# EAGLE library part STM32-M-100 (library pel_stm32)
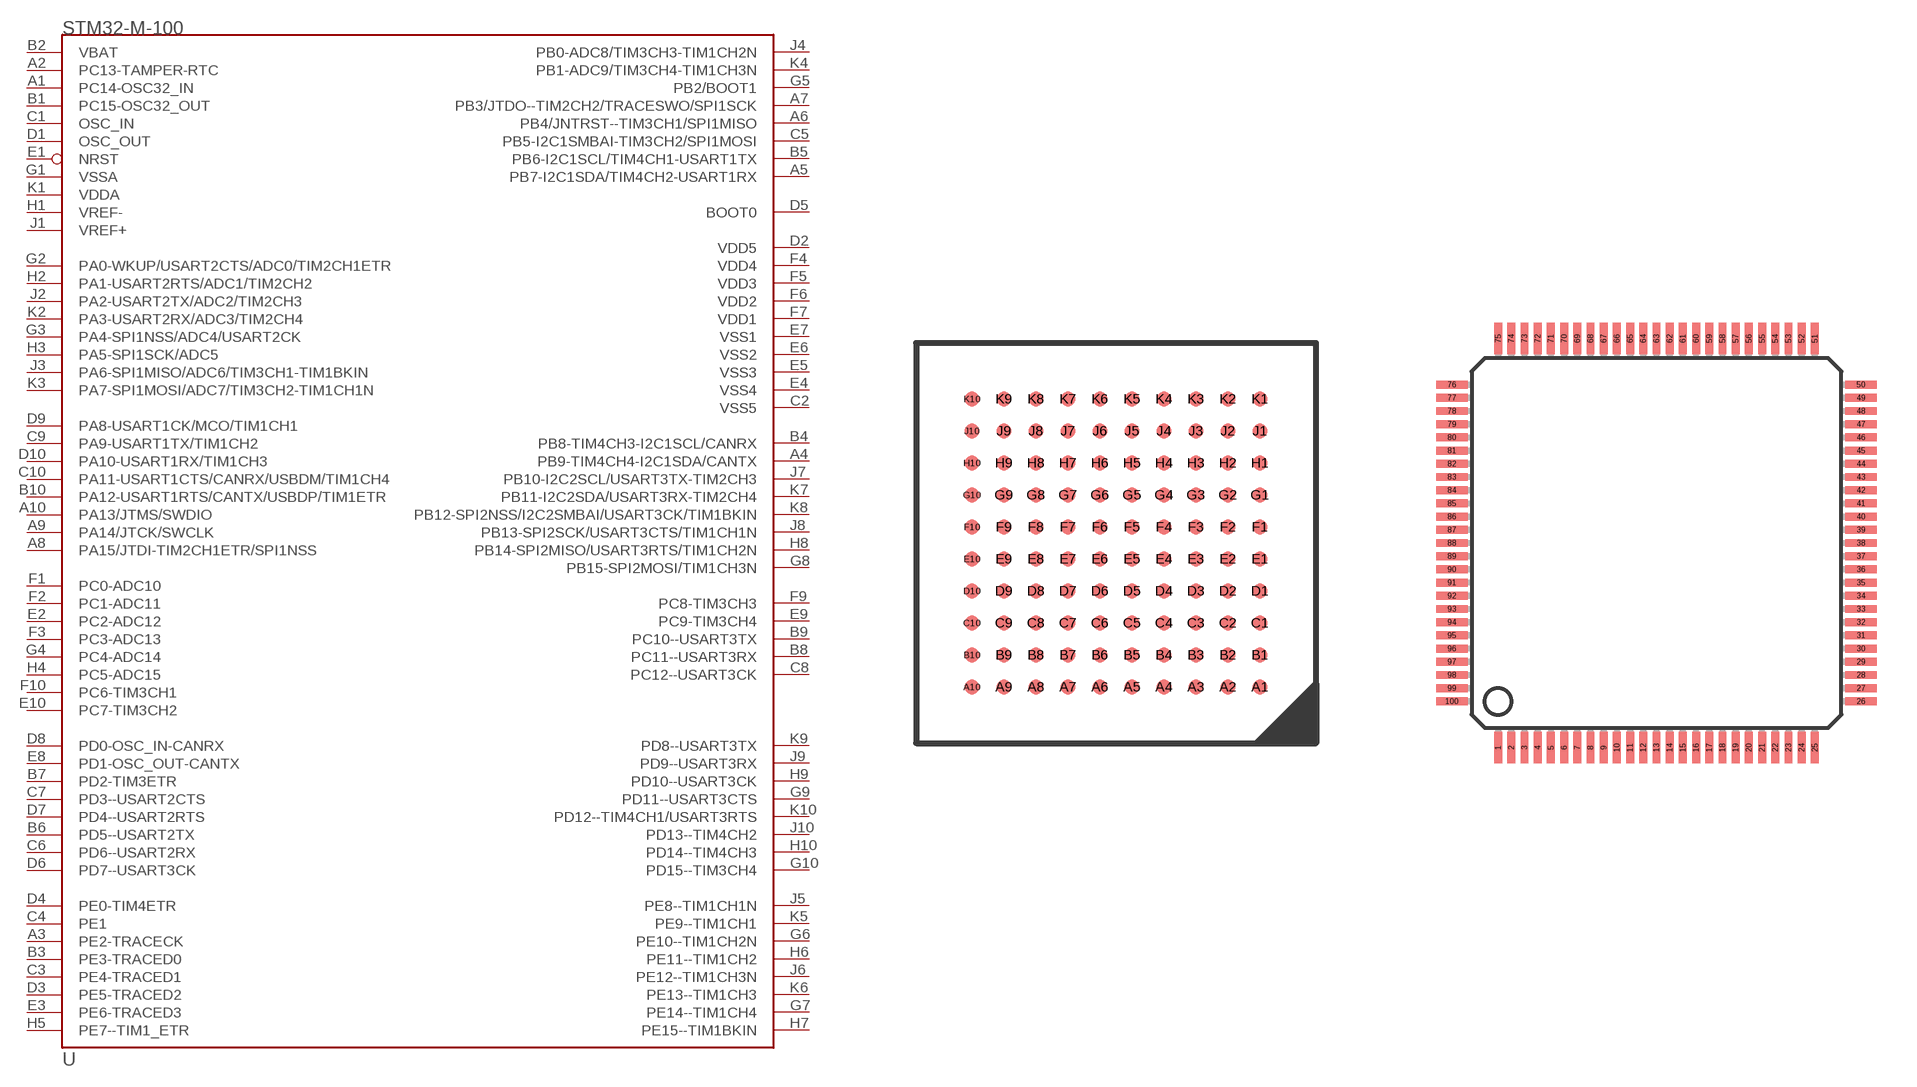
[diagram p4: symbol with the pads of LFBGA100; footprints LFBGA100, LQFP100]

Designator prefix U

## STM32-M-100-LFBGA  [LFBGA100]
A1  PC14-OSC32_IN
A2  PC13-TAMPER-RTC
A3  PE2-TRACECK
A4  PB9-TIM4CH4-I2C1SDA/CANTX
A5  PB7-I2C1SDA/TIM4CH2-USART1RX
A6  PB4/JNTRST--TIM3CH1/SPI1MISO
A7  PB3/JTDO--TIM2CH2/TRACESWO/SPI1SCK
A8  PA15/JTDI-TIM2CH1ETR/SPI1NSS
A9  PA14/JTCK/SWCLK
A10  PA13/JTMS/SWDIO
B1  PC15-OSC32_OUT
B2  VBAT  sup
B3  PE3-TRACED0
B4  PB8-TIM4CH3-I2C1SCL/CANRX
B5  PB6-I2C1SCL/TIM4CH1-USART1TX
B6  PD5--USART2TX
B7  PD2-TIM3ETR
B8  PC11--USART3RX
B9  PC10--USART3TX
B10  PA12-USART1RTS/CANTX/USBDP/TIM1ETR
C1  OSC_IN  in
C2  VSS5
C3  PE4-TRACED1
C4  PE1
C5  PB5-I2C1SMBAI-TIM3CH2/SPI1MOSI
C6  PD6--USART2RX
C7  PD3--USART2CTS
C8  PC12--USART3CK
C9  PA9-USART1TX/TIM1CH2
C10  PA11-USART1CTS/CANRX/USBDM/TIM1CH4
D1  OSC_OUT  out
D2  VDD5
D3  PE5-TRACED2
D4  PE0-TIM4ETR
D5  BOOT0  in
D6  PD7--USART3CK
D7  PD4--USART2RTS
D8  PD0-OSC_IN-CANRX
D9  PA8-USART1CK/MCO/TIM1CH1
D10  PA10-USART1RX/TIM1CH3
E1  NRST
E2  PC2-ADC12
E3  PE6-TRACED3
E4  VSS4
E5  VSS3  sup
E6  VSS2  sup
E7  VSS1  sup
E8  PD1-OSC_OUT-CANTX
E9  PC9-TIM3CH4
E10  PC7-TIM3CH2
F1  PC0-ADC10
F2  PC1-ADC11
F3  PC3-ADC13
F4  VDD4
F5  VDD3  sup
F6  VDD2  sup
F7  VDD1  sup
F9  PC8-TIM3CH3
F10  PC6-TIM3CH1
G1  VSSA  sup
G2  PA0-WKUP/USART2CTS/ADC0/TIM2CH1ETR
G3  PA4-SPI1NSS/ADC4/USART2CK
G4  PC4-ADC14
G5  PB2/BOOT1
G6  PE10--TIM1CH2N
G7  PE14--TIM1CH4
G8  PB15-SPI2MOSI/TIM1CH3N
G9  PD11--USART3CTS
G10  PD15--TIM3CH4
H1  VREF-
H2  PA1-USART2RTS/ADC1/TIM2CH2
H3  PA5-SPI1SCK/ADC5
H4  PC5-ADC15
H5  PE7--TIM1_ETR
H6  PE11--TIM1CH2
H7  PE15--TIM1BKIN
H8  PB14-SPI2MISO/USART3RTS/TIM1CH2N
H9  PD10--USART3CK
H10  PD14--TIM4CH3
J1  VREF+
J2  PA2-USART2TX/ADC2/TIM2CH3
J3  PA6-SPI1MISO/ADC6/TIM3CH1-TIM1BKIN
J4  PB0-ADC8/TIM3CH3-TIM1CH2N
J5  PE8--TIM1CH1N
J6  PE12--TIM1CH3N
J7  PB10-I2C2SCL/USART3TX-TIM2CH3
J8  PB13-SPI2SCK/USART3CTS/TIM1CH1N
J9  PD9--USART3RX
J10  PD13--TIM4CH2
K1  VDDA  sup
K2  PA3-USART2RX/ADC3/TIM2CH4
K3  PA7-SPI1MOSI/ADC7/TIM3CH2-TIM1CH1N
K4  PB1-ADC9/TIM3CH4-TIM1CH3N
K5  PE9--TIM1CH1
K6  PE13--TIM1CH3
K7  PB11-I2C2SDA/USART3RX-TIM2CH4
K8  PB12-SPI2NSS/I2C2SMBAI/USART3CK/TIM1BKIN
K9  PD8--USART3TX
K10  PD12--TIM4CH1/USART3RTS

## STM32-M-100-LQFP  [LQFP100]
1  PE2-TRACECK
2  PE3-TRACED0
3  PE4-TRACED1
4  PE5-TRACED2
5  PE6-TRACED3
6  VBAT  sup
7  PC13-TAMPER-RTC
8  PC14-OSC32_IN
9  PC15-OSC32_OUT
10  VSS5
11  VDD5
12  OSC_IN  in
13  OSC_OUT  out
14  NRST
15  PC0-ADC10
16  PC1-ADC11
17  PC2-ADC12
18  PC3-ADC13
19  VSSA  sup
20  VREF-
21  VREF+
22  VDDA  sup
23  PA0-WKUP/USART2CTS/ADC0/TIM2CH1ETR
24  PA1-USART2RTS/ADC1/TIM2CH2
25  PA2-USART2TX/ADC2/TIM2CH3
26  PA3-USART2RX/ADC3/TIM2CH4
27  VSS4
28  VDD4
29  PA4-SPI1NSS/ADC4/USART2CK
30  PA5-SPI1SCK/ADC5
31  PA6-SPI1MISO/ADC6/TIM3CH1-TIM1BKIN
32  PA7-SPI1MOSI/ADC7/TIM3CH2-TIM1CH1N
33  PC4-ADC14
34  PC5-ADC15
35  PB0-ADC8/TIM3CH3-TIM1CH2N
36  PB1-ADC9/TIM3CH4-TIM1CH3N
37  PB2/BOOT1
38  PE7--TIM1_ETR
39  PE8--TIM1CH1N
40  PE9--TIM1CH1
41  PE10--TIM1CH2N
42  PE11--TIM1CH2
43  PE12--TIM1CH3N
44  PE13--TIM1CH3
45  PE14--TIM1CH4
46  PE15--TIM1BKIN
47  PB10-I2C2SCL/USART3TX-TIM2CH3
48  PB11-I2C2SDA/USART3RX-TIM2CH4
49  VSS1  sup
50  VDD1  sup
51  PB12-SPI2NSS/I2C2SMBAI/USART3CK/TIM1BKIN
52  PB13-SPI2SCK/USART3CTS/TIM1CH1N
53  PB14-SPI2MISO/USART3RTS/TIM1CH2N
54  PB15-SPI2MOSI/TIM1CH3N
55  PD8--USART3TX
56  PD9--USART3RX
57  PD10--USART3CK
58  PD11--USART3CTS
59  PD12--TIM4CH1/USART3RTS
60  PD13--TIM4CH2
61  PD14--TIM4CH3
62  PD15--TIM3CH4
63  PC6-TIM3CH1
64  PC7-TIM3CH2
65  PC8-TIM3CH3
66  PC9-TIM3CH4
67  PA8-USART1CK/MCO/TIM1CH1
68  PA9-USART1TX/TIM1CH2
69  PA10-USART1RX/TIM1CH3
70  PA11-USART1CTS/CANRX/USBDM/TIM1CH4
71  PA12-USART1RTS/CANTX/USBDP/TIM1ETR
72  PA13/JTMS/SWDIO
74  VSS2  sup
75  VDD2  sup
76  PA14/JTCK/SWCLK
77  PA15/JTDI-TIM2CH1ETR/SPI1NSS
78  PC10--USART3TX
79  PC11--USART3RX
80  PC12--USART3CK
81  PD0-OSC_IN-CANRX
82  PD1-OSC_OUT-CANTX
83  PD2-TIM3ETR
84  PD3--USART2CTS
85  PD4--USART2RTS
86  PD5--USART2TX
87  PD6--USART2RX
88  PD7--USART3CK
89  PB3/JTDO--TIM2CH2/TRACESWO/SPI1SCK
90  PB4/JNTRST--TIM3CH1/SPI1MISO
91  PB5-I2C1SMBAI-TIM3CH2/SPI1MOSI
92  PB6-I2C1SCL/TIM4CH1-USART1TX
93  PB7-I2C1SDA/TIM4CH2-USART1RX
94  BOOT0  in
95  PB8-TIM4CH3-I2C1SCL/CANRX
96  PB9-TIM4CH4-I2C1SDA/CANTX
97  PE0-TIM4ETR
98  PE1
99  VSS3  sup
100  VDD3  sup

## Footprint LFBGA100 (pad centres in mm)
smd 0.37 x 0.37: A1 3.6,-3.6; A2 2.8,-3.6; A3 2,-3.6; A4 1.2,-3.6; A5 0.4,-3.6; A6 -0.4,-3.6; A7 -1.2,-3.6; A8 -2,-3.6; A9 -2.8,-3.6; A10 -3.6,-3.6; B1 3.6,-2.8; B2 2.8,-2.8; B3 2,-2.8; B4 1.2,-2.8; B5 0.4,-2.8; B6 -0.4,-2.8; B7 -1.2,-2.8; B8 -2,-2.8; B9 -2.8,-2.8; B10 -3.6,-2.8; C1 3.6,-2; C2 2.8,-2; C3 2,-2; C4 1.2,-2; C5 0.4,-2; C6 -0.4,-2; C7 -1.2,-2; C8 -2,-2; C9 -2.8,-2; C10 -3.6,-2; D1 3.6,-1.2; D2 2.8,-1.2; D3 2,-1.2; D4 1.2,-1.2; D5 0.4,-1.2; D6 -0.4,-1.2; D7 -1.2,-1.2; D8 -2,-1.2; D9 -2.8,-1.2; D10 -3.6,-1.2; E1 3.6,-0.4; E2 2.8,-0.4; E3 2,-0.4; E4 1.2,-0.4; E5 0.4,-0.4; E6 -0.4,-0.4; E7 -1.2,-0.4; E8 -2,-0.4; E9 -2.8,-0.4; E10 -3.6,-0.4; F1 3.6,0.4; F2 2.8,0.4; F3 2,0.4; F4 1.2,0.4; F5 0.4,0.4; F6 -0.4,0.4; F7 -1.2,0.4; F8 -2,0.4; F9 -2.8,0.4; F10 -3.6,0.4; G1 3.6,1.2; G2 2.8,1.2; G3 2,1.2; G4 1.2,1.2; G5 0.4,1.2; G6 -0.4,1.2; G7 -1.2,1.2; G8 -2,1.2; G9 -2.8,1.2; G10 -3.6,1.2; H1 3.6,2; H2 2.8,2; H3 2,2; H4 1.2,2; H5 0.4,2; H6 -0.4,2; H7 -1.2,2; H8 -2,2; H9 -2.8,2; H10 -3.6,2; J1 3.6,2.8; J2 2.8,2.8; J3 2,2.8; J4 1.2,2.8; J5 0.4,2.8; J6 -0.4,2.8; J7 -1.2,2.8; J8 -2,2.8; J9 -2.8,2.8; J10 -3.6,2.8; K1 3.6,3.6; K2 2.8,3.6; K3 2,3.6; K4 1.2,3.6; K5 0.4,3.6; K6 -0.4,3.6; K7 -1.2,3.6; K8 -2,3.6; K9 -2.8,3.6; K10 -3.6,3.6

## Footprint LQFP100 (pad centres in mm)
smd 0.3 x 1.2: 1 -6,-7.75; 2 -5.5,-7.75; 3 -5,-7.75; 4 -4.5,-7.75; 5 -4,-7.75; 6 -3.5,-7.75; 7 -3,-7.75; 8 -2.5,-7.75; 9 -2,-7.75; 10 -1.5,-7.75; 11 -1,-7.75; 12 -0.5,-7.75; 13 0,-7.75; 14 0.5,-7.75; 15 1,-7.75; 16 1.5,-7.75; 17 2,-7.75; 18 2.5,-7.75; 19 3,-7.75; 20 3.5,-7.75; 21 4,-7.75; 22 4.5,-7.75; 23 5,-7.75; 24 5.5,-7.75; 25 6,-7.75; 51 6,7.75; 52 5.5,7.75; 53 5,7.75; 54 4.5,7.75; 55 4,7.75; 56 3.5,7.75; 57 3,7.75; 58 2.5,7.75; 59 2,7.75; 60 1.5,7.75; 61 1,7.75; 62 0.5,7.75; 63 0,7.75; 64 -0.5,7.75; 65 -1,7.75; 66 -1.5,7.75; 67 -2,7.75; 68 -2.5,7.75; 69 -3,7.75; 70 -3.5,7.75; 71 -4,7.75; 72 -4.5,7.75; 73 -5,7.75; 74 -5.5,7.75; 75 -6,7.75
smd 1.2 x 0.3: 26 7.75,-6; 27 7.75,-5.5; 28 7.75,-5; 29 7.75,-4.5; 30 7.75,-4; 31 7.75,-3.5; 32 7.75,-3; 33 7.75,-2.5; 34 7.75,-2; 35 7.75,-1.5; 36 7.75,-1; 37 7.75,-0.5; 38 7.75,0; 39 7.75,0.5; 40 7.75,1; 41 7.75,1.5; 42 7.75,2; 43 7.75,2.5; 44 7.75,3; 45 7.75,3.5; 46 7.75,4; 47 7.75,4.5; 48 7.75,5; 49 7.75,5.5; 50 7.75,6; 76 -7.75,6; 77 -7.75,5.5; 78 -7.75,5; 79 -7.75,4.5; 80 -7.75,4; 81 -7.75,3.5; 82 -7.75,3; 83 -7.75,2.5; 84 -7.75,2; 85 -7.75,1.5; 86 -7.75,1; 87 -7.75,0.5; 88 -7.75,0; 89 -7.75,-0.5; 90 -7.75,-1; 91 -7.75,-1.5; 92 -7.75,-2; 93 -7.75,-2.5; 94 -7.75,-3; 95 -7.75,-3.5; 96 -7.75,-4; 97 -7.75,-4.5; 98 -7.75,-5; 99 -7.75,-5.5; 100 -7.75,-6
